| IBIS file generated by GenIBIS.pl Version 2.11
|   omap3530cbc
[IBIS ver]   4.1
[File name]   sprm323.ibs
[File Rev]   1.0
[Date]   Thu Dec 10, 2009, 9:15:0
[Source]   Data created at Texas Instruments
[Notes]   1) Model checked with IBISCHK4 and contains...
   16 errors relating to DC endpoints. These errors can be waived
   and relate to special modelling of active feedback IOs.
   180 warnings relating to non-monotonic behavior, non-zero
   GND/POWER Clamp values and C_comp max/min values. These
   warnings can be waived.
[Disclaimer] Please be aware that in the absence of a written agreement,
   Texas Instruments (TI) assumes no liability for: 1) the
   accuracy of the IBIS models provided to your company, 2) the
   proper functioning of these IBIS models in your design or for
   any resulting applications, or, 3) infringement of patents,
   copyrights, or intellectual property rights resulting from
   your use of these IBIS models. TI provides IBIS models as a
   service to our customers and therefore reserves the right to
   limit distribution of the IBIS models.
[Copyright]   Property of Texas Instruments Incorporated. Unauthorised
   reproduction and/or distribution is strictly prohibited. This
   product is protected under copyright law and trade secret law
   as an unpublished work. Created 1999,(C) Copyright 1999-2001,
   Texas Instruments Incorporated., All Rights Reserved. These
   commodities are under the U.S. Government distribution license
   control.As such,they are not to be re-exported without the
   prior approval of the U.S. Department of Commerce.
|   Component omap3530cbc
[Component]   omap3530cbc
[Manufacturer]   Texas Instruments.
[Package]
|   typ   min   max
R_pkg   1.24535   3.07E-2   2.46E0
L_pkg   4.9035E-009   3.77E-10   9.43E-9
C_pkg   1.941E-012   5.72E-13   3.31E-12
[Pin]   signal_name   model_name   R_pin   L_pin   C_pin
A3   gpmc_ncs2   Selector16   7.47E-1   2.93E-9   1.21E-12
A24   cam_d2   Selector12   6.25E-1   3.26E-9   1.31E-12
AA1   gpmc_d1   Selector16   1.96E0   8.19E-9   3.09E-12
AA2   gpmc_d0   Selector16   1.81E0   7.48E-9   3.08E-12
AA3   etk_d3   Selector16   6.29E-1   3.01E-9   1.20E-12
AA4   etk_d8   Selector1   8.17E-1   3.80E-9   1.32E-12
AA24   uart2_rts   Selector23   2.77E-1   2.00E-9   9.98E-13
AA25   dss_data12   Selector24   3.83E-1   1.97E-9   1.03E-12
AB1   etk_d5   Selector1   6.42E-1   3.90E-9   1.49E-12
AB2   etk_clk   Selector16   7.57E-1   3.49E-9   1.17E-12
AB4   i2c3_scl   Selector7   8.04E-1   3.18E-9   1.54E-12
AB25   dss_data23   Selector24   3.95E-1   2.43E-9   7.96E-13
AB26   dss_data15   Selector24   3.76E-1   2.32E-9   1.19E-12
AC1   gpmc_d3   Selector16   2.44E0   9.43E-9   3.17E-12
AC3   etk_d0   Selector16   7.48E-1   3.54E-9   1.20E-12
AC4   i2c3_sda   Selector7   4.25E-1   1.96E-9   1.16E-12
AC6   gpmc_nwp   Selector1   1.90E0   7.54E-9   3.00E-12
AC8   gpmc_wait1   Selector16   1.77E0   6.52E-9   2.93E-12
AC11   gpmc_wait0   Selector26   1.56E0   5.94E-9   2.85E-12
AC25   dss_data22   Selector24   3.90E-1   2.06E-9   9.02E-13
AC26   dss_data10   Selector24   4.20E-1   2.22E-9   1.12E-12
AD1   gpmc_ncs1   Selector16   2.18E0   9.09E-9   3.27E-12
AD3   etk_d2   Selector16   7.54E-1   3.54E-9   1.19E-12
AD5   gpmc_d6   Selector16   2.12E0   8.02E-9   3.26E-12
AD6   gpmc_d5   Selector16   1.82E0   7.47E-9   2.93E-12
AD7   sys_nreswarm   Selector25   5.19E-1   2.57E-9   2.06E-12
AD8   gpmc_ncs0   Selector11   1.84E0   6.93E-9   3.12E-12
AD16   gpio_113   Selector9   3.55E-1   1.79E-9   1.04E-12
AD17   gpio_112   Selector31   3.06E-1   1.92E-9   1.09E-12
AD21   uart2_rx   Selector23   2.39E-1   1.71E-9   9.84E-13
AD23   dss_data4   Model19   7.20E-1   2.65E-9   1.21E-12
AD24   dss_data5   Model19   6.03E-1   2.55E-9   1.08E-12
AD26   dss_data11   Selector24   4.78E-1   2.34E-9   1.08E-12
AE3   etk_d6   Selector1   9.02E-1   4.42E-9   1.31E-12
AE4   etk_d10   Selector1   8.76E-1   4.69E-9   1.67E-12
AE6   etk_d12   Selector1   7.45E-1   3.29E-9   1.36E-12
AE9   etk_d15   Selector1   4.16E-1   2.87E-9   1.34E-12
AE14   sys_clkout1   Selector5   7.36E-1   3.62E-9   1.65E-12
AE15   cam_d1   Selector3   1.92E-1   1.75E-9   9.80E-13
AE16   cam_d0   Selector20   1.57E-1   1.38E-9   9.16E-13
AE17   gpio_115   Selector32   3.17E-1   2.36E-9   1.04E-12
AE21   dss_data0   Model19   5.10E-1   2.83E-9   1.42E-12
AE23   dss_data2   Model19   4.99E-1   3.29E-9   1.11E-12
A23   cam_wen   Selector1   5.52E-1   3.42E-9   1.33E-12
AA26   dss_data14   Selector24   3.46E-1   1.74E-9   1.04E-12
AB3   etk_ctl   Selector16   6.33E-1   3.04E-9   1.35E-12
AC2   gpmc_d2   Selector16   2.46E0   8.74E-9   3.20E-12
AC5   gpmc_d7   Selector16   1.91E0   7.35E-9   3.03E-12
AD2   etk_d7   Selector1   8.44E-1   4.04E-9   1.21E-12
AD4   etk_d1   Selector1   8.44E-1   3.97E-9   1.36E-12
AD10   gpmc_nadv_ale   Selector22   1.79E0   7.57E-9   3.16E-12
AD15   i2c4_scl   Selector21   4.33E-1   2.80E-9   1.29E-12
AD22   uart2_tx   Selector23   3.75E-1   2.44E-9   1.11E-12
AE5   gpmc_d4   Selector16   1.96E0   7.81E-9   3.31E-12
AE18   gpio_114   Selector13   3.09E-1   2.36E-9   9.80E-13
AE20   sys_32k   Model94   1.18E0   6.31E-9   2.27E-12
AE22   dss_data1   Model19   4.68E-1   2.77E-9   1.32E-12
AE24   dss_data3   Model19   6.80E-1   3.18E-9   1.27E-12
AF6   etk_d11   Selector1   1.02E0   4.26E-9   1.32E-12
AF7   etk_d13   Selector1   1.17E0   5.30E-9   1.75E-12
AF9   etk_d14   Selector1   5.90E-1   3.89E-9   1.47E-12
AF19   sys_xtalin   Model82   7.18E-1   3.00E-9   1.26E-12
B3   gpmc_wait2   Selector16   7.66E-1   3.69E-9   1.31E-12
B4   gpmc_ncs4   Selector16   5.76E-1   3.21E-9   1.17E-12
B5   gpmc_ncs6   Selector16   6.68E-1   3.19E-9   1.21E-12
B6   gpmc_ncs3   Selector16   6.49E-1   2.82E-9   1.30E-12
B23   cam_fld   Selector1   4.18E-1   2.91E-9   1.11E-12
B24   cam_d3   Selector12   5.18E-1   2.76E-9   1.16E-12
C1   i2c2_sda   Selector7   1.72E0   6.60E-9   2.51E-12
C2   i2c2_scl   Selector7   1.54E0   6.33E-9   2.44E-12
C3   sys_boot2   Selector18   1.50E0   6.37E-9   2.20E-12
C4   gpmc_ncs5   Selector16   6.97E-1   3.53E-9   1.21E-12
C5   gpmc_ncs7   Selector16   4.85E-1   2.50E-9   1.27E-12
C6   gpmc_wait3   Selector16   4.60E-1   2.30E-9   1.21E-12
C23   cam_hs   Selector1   3.12E-1   2.16E-9   1.04E-12
C24   cam_d5   Selector12   5.71E-1   2.36E-9   1.16E-12
C25   cam_xclka   Selector1   5.14E-1   2.85E-9   1.05E-12
C26   cam_pclk   Selector1   5.65E-1   3.44E-9   1.23E-12
D1   gpmc_a9   Selector16   9.12E-1   4.13E-9   1.74E-12
D2   gpmc_a10   Selector16   5.01E-1   3.27E-9   1.44E-12
D3   sys_boot1   Selector18   1.64E0   6.91E-9   2.73E-12
D4   sys_boot6   Selector18   1.47E0   5.94E-9   2.63E-12
D23   cam_vs   Selector1   3.72E-1   2.45E-9   1.11E-12
D24   cam_d4   Selector12   4.53E-1   1.78E-9   1.04E-12
D25   cam_d10   Selector12   5.59E-1   2.67E-9   1.09E-12
D26   cam_strobe   Selector1   5.32E-1   3.02E-9   1.07E-12
E1   gpmc_a7   Selector16   7.35E-1   4.07E-9   1.41E-12
E2   gpmc_a8   Selector16   4.80E-1   3.15E-9   1.28E-12
E3   sys_boot3   Selector18   1.51E0   6.23E-9   2.64E-12
E4   sys_boot4   Selector18   1.35E0   5.60E-9   2.40E-12
E25   cam_xclkb   Selector1   4.33E-1   2.69E-9   9.49E-13
E26   cam_d11   Selector1   4.59E-1   2.76E-9   9.36E-13
F1   gpmc_a5   Selector1   8.42E-1   4.22E-9   1.51E-12
F2   gpmc_a6   Selector16   7.94E-1   3.87E-9   1.47E-12
F3   sys_boot0   Selector18   1.45E0   5.48E-9   2.37E-12
F23   uart3_cts_rctx   Selector23   3.29E-1   1.68E-9   1.11E-12
F24   uart3_rts_sd   Selector23   2.70E-1   1.77E-9   9.83E-13
F25   dss_data20   Selector2   5.35E-1   2.94E-9   9.30E-13
F26   dss_acbias   Selector8   5.81E-1   3.51E-9   1.15E-12
G2   gpmc_a4   Selector1   7.36E-1   4.12E-9   1.56E-12
G3   sys_boot5   Selector18   1.32E0   5.19E-9   2.07E-12
G24   uart3_tx_irtx   Selector23   3.45E-1   2.18E-9   1.00E-12
G25   dss_pclk   Selector2   3.63E-1   2.24E-9   8.87E-13
G26   dss_data6   Selector8   3.96E-1   2.81E-9   1.10E-12
H1   gpmc_a2   Selector1   1.04E0   4.79E-9   1.82E-12
H2   gpmc_a3   Selector1   8.67E-1   4.11E-9   1.60E-12
H3   uart1_rx   Selector1   1.06E0   3.86E-9   1.47E-12
H24   uart3_rx_irrx   Selector23   2.90E-1   1.95E-9   6.96E-13
H25   dss_data7   Selector8   4.05E-1   2.79E-9   9.14E-13
H26   dss_data8   Selector8   4.43E-1   2.90E-9   9.44E-13
J1   gpmc_nbe1   Selector1   1.12E0   5.06E-9   1.81E-12
J2   gpmc_a1   Selector1   1.01E0   4.83E-9   1.80E-12
J23   hdq_sio   Selector23   1.45E-1   1.42E-9   1.13E-12
J24   i2c1_sda   Selector4   3.24E-1   2.10E-9   9.83E-13
J25   i2c1_scl   Selector4   1.15E-1   1.35E-9   8.80E-13
J26   dss_data9   Selector8   4.62E-1   3.03E-9   9.58E-13
K2   gpmc_nbe0_cle   Selector1   9.96E-1   4.57E-9   1.82E-12
K3   mmc2_dat7   Selector1   1.24E0   6.44E-9   2.30E-12
K18   mmc1_dat2   Selector28   2.94E-1   2.34E-9   1.22E-12
K24   dss_hsync   Selector2   2.27E-1   1.57E-9   8.73E-13
L2   gpmc_d14   Selector16   3.82E-1   2.10E-9   1.19E-12
L3   mmc2_dat6   Selector1   6.40E-1   2.77E-9   1.14E-12
L4   uart1_tx   Selector10   6.79E-1   3.49E-9   1.88E-12
L18   mmc1_cmd   Selector28   2.79E-1   2.17E-9   9.60E-13
L25   dss_data16   Selector8   2.53E-1   1.30E-9   8.13E-13
L26   dss_data17   Selector8   4.54E-1   3.09E-9   1.09E-12
M1   gpmc_nwe   Selector11   4.67E-1   2.17E-9   1.19E-12
M2   gpmc_d15   Selector16   3.28E-1   1.78E-9   1.03E-12
M3   mmc2_dat5   Selector1   7.43E-1   4.22E-9   1.96E-12
M18   mmc1_dat1   Selector28   2.82E-1   1.81E-9   9.77E-13
M19   mmc1_dat0   Selector28   2.13E-1   1.61E-9   6.88E-13
M20   mmc1_dat4   Selector6   1.99E-1   1.66E-9   8.17E-13
M24   dss_data18   Selector8   3.27E-1   1.44E-9   8.69E-13
M25   dss_vsync   Selector2   3.10E-1   2.18E-9   1.10E-12
M26   dss_data19   Selector8   3.90E-1   2.24E-9   8.08E-13
N1   gpmc_clk   Selector1   7.04E-1   3.92E-9   1.73E-12
N2   gpmc_noe   Selector11   6.04E-1   2.69E-9   1.24E-12
N3   mcbsp3_dr   Selector1   5.26E-1   2.45E-9   1.07E-12
N19   mmc1_clk   Selector28   1.45E-1   1.74E-9   9.13E-13
N20   mmc1_dat3   Selector28   1.01E-1   1.19E-9   6.33E-13
N24   dss_data21   Selector8   4.35E-1   2.40E-9   9.99E-13
N25   cam_d8   Selector15   4.37E-1   2.49E-9   9.27E-13
N26   cam_d9   Selector17   3.55E-1   2.45E-9   9.81E-13
P1   gpmc_d13   Selector16   7.40E-1   4.30E-9   2.00E-12
P3   mcbsp3_dx   Selector1   4.51E-1   2.01E-9   9.47E-13
P7   mcspi1_somi   Selector14   4.61E-1   2.36E-9   1.03E-12
P8   mcspi1_simo   Selector14   3.00E-1   1.40E-9   7.95E-13
P9   mcspi1_clk   Selector14   3.47E-1   1.85E-9   7.54E-13
P17   mmc1_dat5   Selector6   3.28E-1   2.48E-9   1.39E-12
P18   mmc1_dat6   Selector6   2.59E-1   2.33E-9   9.77E-13
P19   mmc1_dat7   Selector6   1.89E-1   1.93E-9   7.54E-13
P20   mcbsp1_fsx   Selector1   2.37E-1   2.33E-9   9.07E-13
P25   cam_d6   Selector19   4.93E-1   1.98E-9   1.12E-12
P26   cam_d7   Selector30   4.82E-1   2.37E-9   8.33E-13
R2   uart1_rts   Selector10   3.09E-1   2.17E-9   9.35E-13
R3   mcbsp4_dx   Selector1   1.02E-1   1.66E-9   9.81E-13
R7   mcspi1_cs0   Selector14   2.61E-1   1.49E-9   6.48E-13
R8   mcspi1_cs1   Selector14   2.71E-1   1.44E-9   1.66E-12
R9   mcspi1_cs2   Selector14   3.46E-1   2.20E-9   9.66E-13
R10   mmc2_cmd   Selector16   4.22E-1   2.14E-9   8.09E-13
R18   mcbsp2_clkx   Selector14   2.60E-1   2.11E-9   8.58E-13
R19   mcbsp2_dx   Selector14   1.96E-1   1.82E-9   7.11E-13
T1   gpmc_d10   Selector16   1.14E0   5.46E-9   2.19E-12
T3   mcbsp4_fsx   Selector1   4.59E-1   2.81E-9   1.34E-12
T8   mcspi1_cs3   Selector16   3.46E-1   1.61E-9   1.72E-12
T9   mmc2_dat1   Selector16   4.08E-1   2.06E-9   8.68E-13
T10   mmc2_dat0   Selector16   3.34E-1   1.94E-9   8.12E-13
T17   mcbsp1_clkx   Selector1   3.41E-1   2.70E-9   9.99E-13
T18   mcbsp2_dr   Selector14   3.68E-1   2.37E-9   8.89E-13
T19   mcbsp_clks   Selector1   2.58E-1   1.71E-9   8.20E-13
T20   mcbsp1_dr   Selector1   2.70E-1   1.42E-9   6.81E-13
U1   gpmc_d12   Selector16   5.96E-1   3.80E-9   1.80E-12
U2   gpmc_d11   Selector16   1.27E0   5.73E-9   2.38E-12
U3   mcbsp3_clkx   Selector1   1.39E-1   1.67E-9   9.93E-13
U4   mcbsp4_dr   Selector12   2.59E-1   1.82E-9   1.04E-12
U8   mcspi2_somi   Selector1   6.06E-1   3.40E-9   1.49E-12
U9   mmc2_dat3   Selector16   4.96E-1   2.56E-9   1.08E-12
U10   mmc2_dat2   Selector16   5.08E-1   2.50E-9   1.16E-12
U15   jtag_ntrst   Selector27   6.11E-1   2.84E-9   8.87E-13
U16   jtag_tdi   Model71   5.29E-1   2.78E-9   8.93E-13
U17   mcbsp1_dx   Selector1   3.09E-1   2.47E-9   1.12E-12
U18   mcbsp2_fsx   Selector14   3.54E-1   2.31E-9   9.48E-13
U19   mcbsp1_clkr   Selector1   1.73E-1   1.70E-9   8.85E-13
U20   hsusb0_stp   Selector16   3.12E-1   1.58E-9   8.48E-13
V1   gpmc_d8   Selector16   1.46E0   6.54E-9   2.46E-12
V2   etk_d9   Selector1   3.29E-1   2.50E-9   8.29E-13
V3   mcbsp4_clkx   Selector1   3.99E-1   2.11E-9   9.74E-13
V8   mcspi2_cs0   Selector16   6.63E-1   3.57E-9   1.54E-12
V9   mcspi2_cs1   Selector1   6.34E-1   3.43E-9   1.61E-12
V10   mmc2_dat4   Selector1   5.69E-1   3.58E-9   1.27E-12
V12   sys_off_mode   Selector25   3.46E-1   2.02E-9   1.08E-12
V13   sys_nrespwron   Model75   4.08E-1   2.14E-9   1.23E-12
V14   jtag_tck   Selector27   5.65E-1   2.77E-9   1.19E-12
V15   jtag_tms_tmsc   Selector29   5.43E-1   2.65E-9   9.97E-13
V16   sys_nirq   Selector23   2.09E-1   1.36E-9   8.78E-13
V17   mcbsp1_fsr   Selector1   3.07E-1   2.49E-9   1.13E-12
V18   hsusb0_data2   Selector1   2.94E-1   2.26E-9   9.31E-13
V19   hsusb0_dir   Selector1   2.87E-1   2.14E-9   1.03E-12
V20   hsusb0_data0   Selector1   2.73E-1   1.93E-9   7.84E-13
W2   uart1_cts   Selector12   3.42E-1   2.38E-9   9.23E-13
W3   mcbsp3_fsx   Selector1   3.64E-1   2.41E-9   1.02E-12
W7   mcspi2_clk   Selector1   5.48E-1   3.09E-9   1.19E-12
W8   mcspi2_simo   Selector1   7.07E-1   3.59E-9   1.50E-12
W10   mmc2_clk   Selector1   7.12E-1   4.00E-9   1.41E-12
W11   sys_clkout2   Selector1   1.72E-1   1.25E-9   9.43E-13
W13   jtag_rtck   Selector5   3.45E-1   2.12E-9   1.05E-12
W15   sys_clkreq   Selector25   2.67E-1   1.84E-9   8.88E-13
W16   i2c4_sda   Selector21   4.99E-1   2.44E-9   1.05E-12
W17   hsusb0_data4   Selector1   3.42E-1   2.23E-9   9.95E-13
W18   hsusb0_nxt   Selector1   2.37E-1   2.31E-9   9.78E-13
W19   hsusb0_clk   Selector1   4.24E-1   2.66E-9   9.02E-13
W20   hsusb0_data3   Selector1   1.50E-1   1.53E-9   6.88E-13
Y1   gpmc_d9   Selector16   1.59E0   7.11E-9   2.51E-12
Y3   etk_d4   Selector1   2.31E-1   1.56E-9   1.06E-12
Y13   jtag_tdo   Selector5   2.38E-1   1.32E-9   7.11E-13
Y14   jtag_emu1   Selector23   3.98E-1   2.16E-9   1.04E-12
Y15   jtag_emu0   Selector23   3.66E-1   1.99E-9   1.18E-12
Y17   hsusb0_data7   Selector1   5.56E-1   3.27E-9   1.03E-12
Y18   hsusb0_data5   Selector1   3.07E-1   2.39E-9   8.93E-13
Y19   hsusb0_data6   Selector1   3.56E-1   2.10E-9   7.98E-13
Y20   hsusb0_data1   Selector1   2.07E-1   1.97E-9   8.03E-13
Y24   uart2_cts   Selector23   3.69E-1   2.25E-9   1.26E-12
Y25   dss_data13   Selector24   3.72E-1   1.81E-9   9.39E-13
| Device pads which are not required to be modeled. Included for completeness
|A18   vdds
|AB24   vdds_sdi
|AC7   vdds
|AC15   vdds
|AC18   vdds
|AC19   vss_dsi
|AC21   vdd_core
|AC24   vdds
|AD18   vdds_csi2
|AD20   vdds
|AE10   vdds
|AE19   cap_vdd_dsi
|AC16   vss_csi2
|AD19   vdds_dsi
|AF20   sys_xtalout   BQ0073VDDUS.4
|C11   vdds
|D5   vpp
|D9   vdds
|D13   vdd_mpu_iva
|D15   vdd_core
|E24   vdds
|G4   vdds
|G9   vdd_mpu_iva
|G11   vdd_core
|G12   vdd_mpu_iva
|G18   vdd_core
|H7   vdd_mpu_iva
|H20   vdd_core
|J15   vdds
|J18   vdds
|K11   vdd_mpu_iva
|L7   vdds
|L9   vdd_mpu_iva
|L19   vss_csib
|L20   vdds_csib
|L24   vdds
|M4   vdds
|M7   vdd_core
|M9   vdd_mpu_iva
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[Model Selector] Selector1
Model4 1.8V-I/O-X-SLOW
Model5 1.8V-I/O-X-FAST
Model6 1.8V-INPUT-PD-X
Model7 1.8V-INPUT-PI-X
Model8 1.8V-INPUT-PU-X
| Model selector for model set 1,2,3
|   Usage O#1.8V#PD/PI/PU##BQ0232CS_7LM
[Model Selector] Selector2
Model1 1.8V-I/O-PD-X
Model2 1.8V-I/O-PI-X
Model3 1.8V-I/O-PU-X
| Model selector for model set 10,9
|   Usage I#1.8V###CSI2PHY3LANE_7LM.8
[Model Selector] Selector3
Model10 1.8V-INPUT-X-X-GPI mode
Model9 1.8V-INPUT-X-X-LPRX Mode
| Model selector for model set 11,12
|   Usage IOOD#1.8V#PD/PI/PU##BQ0246S_7LM
[Model Selector] Selector4
Model11 1.8000V-I/O_OPEN_DRAIN-X-STANDARD
Model12 1.8000V-I/O_OPEN_DRAIN-X-LOWC
| Model selector for model set 13,14,15
|   Usage O#1.8V###BQ0253CS_7LM
[Model Selector] Selector5
Model13 1.8V-I/O-PD-X
Model14 1.8V-I/O-PI-X
Model15 1.8V-I/O-PU-X
| Model selector for model set 16,17,18
|   Usage IO#1.8V#PD/PI/PU##BQ0447S_7LM
[Model Selector] Selector6
Model16 1.8V-I/O-PD-X
Model17 1.8V-I/O-PI-X
Model18 1.8V-I/O-PU-X
| Model selector for model set 11,12,23,24
|   Usage IO#1.8V#PD/PI/PU##BQ0246S_7LM
|   IOOD#1.8V#PD/PI/PU##BQ0246S_7LM
[Model Selector] Selector7
Model11 1.8000V-I/O_OPEN_DRAIN-X-STANDARD
Model12 1.8000V-I/O_OPEN_DRAIN-X-LOWC
Model23 1.8000V-I/O-X-X
Model24 1.8000V-I/O-X-HIGHC
| Model selector for model set 20,21,22
|   Usage O#1.8V#PD/PI/PU##BQ0230CS_7LM
[Model Selector] Selector8
Model20 1.8V-I/O-PD-X
Model21 1.8V-I/O-PI-X
Model22 1.8V-I/O-PU-X
| Model selector for model set 25,26
|   Usage I#1.8V###CSI2PHY3LANE_7LM.4
[Model Selector] Selector9
Model25 1.8V-INPUT-X-X-LPRX Mode
Model26 1.8V-INPUT-X-X-GPI mode
| Model selector for model set 4,5
|   Usage O#1.8V#PD/PI/PU##BQ0267CS_7LM
[Model Selector] Selector10
Model4 1.8V-I/O-X-SLOW
Model5 1.8V-I/O-X-FAST
| Model selector for model set 27,28
|   Usage O#1.8V#PD/PI/PU##OQ0164CS_7LM
[Model Selector] Selector11
Model27 1.8V-3-STATE-X-SLOW
Model28 1.8V-3-STATE-X-FAST
| Model selector for model set 6,7,8
|   Usage I#1.8V#PD/PI/PU##BQ0267CS_7LM
[Model Selector] Selector12
Model6 1.8V-INPUT-PD-X
Model7 1.8V-INPUT-PI-X
Model8 1.8V-INPUT-PU-X
| Model selector for model set 29,30
|   Usage I#1.8V###CSI2PHY3LANE_7LM.5
[Model Selector] Selector13
Model29 1.8V-INPUT-X-X-LPRX Mode
Model30 1.8V-INPUT-X-X-GPI mode
| Model selector for model set 31,32,33,34,35,36,37,38,39,40,41,42
|   Usage O#1.8V#PD/PI/PU##BQOMAPPROGIOCSHYFBPB_7LM
[Model Selector] Selector14
Model31 1.8V-I/O-PD-DS00
Model32 1.8V-I/O-PD-DS11
Model33 1.8V-I/O-PD-DS10
Model34 1.8V-I/O-PD-DS01
Model35 1.8V-I/O-PI-DS11
Model36 1.8V-I/O-PI-DS10
Model37 1.8V-I/O-PI-DS01
Model38 1.8V-I/O-PI-DS00
Model39 1.8V-I/O-PU-DS00
Model40 1.8V-I/O-PU-DS11
Model41 1.8V-I/O-PU-DS10
Model42 1.8V-I/O-PU-DS01
| Model selector for model set 43,44,45
|   Usage I#1.8V#PD/PI/PU##CCPV2_7LM.3
[Model Selector] Selector15
Model43 1.8V-I/O-PD-X
Model44 1.8V-I/O-PI-X
Model45 1.8V-I/O-PU-X
| Model selector for model set 46,47,48,49,50
|   Usage IO#1.8V#PD/PI/PU##BQ0268CS_7LM
|   O#1.8V#PD/PU##BQ0268CS_7LM
[Model Selector] Selector16
Model46 1.8V-I/O-X-SLOW
Model47 1.8V-I/O-X-FAST
Model48 1.8V-INPUT-PD-X
Model49 1.8V-INPUT-PI-X
Model50 1.8V-INPUT-PU-X
| Model selector for model set 51,52,53
|   Usage I#1.8V#PD/PI/PU##CCPV2_7LM.4
[Model Selector] Selector17
Model51 1.8V-I/O-PD-X
Model52 1.8V-I/O-PI-X
Model53 1.8V-I/O-PU-X
| Model selector for model set 54,55,56
|   Usage IO#1.8V#PD/PI/PU##BQ0228CS_7LM
[Model Selector] Selector18
Model54 1.8V-I/O-PD-X
Model55 1.8V-I/O-PI-X
Model56 1.8V-I/O-PU-X
| Model selector for model set 57,58,59
|   Usage I#1.8V#PD/PI/PU##CCPV2_7LM.1
[Model Selector] Selector19
Model57 1.8V-I/O-PD-X
Model58 1.8V-I/O-PI-X
Model59 1.8V-I/O-PU-X
| Model selector for model set 60,61
|   Usage I#1.8V###CSI2PHY3LANE_7LM.7
[Model Selector] Selector20
Model60 1.8V-INPUT-X-X-LPRX Mode
Model61 1.8V-INPUT-X-X-GPI mode
| Model selector for model set 62,63,64,65
|   Usage IOOD#1.8V#PD/PI/PU##BQ0245S_7LM
|   O#1.8V#PD/PI/PU##BQ0245S_7LM
[Model Selector] Selector21
Model62 1.8000V-I/O_OPEN_DRAIN-X-STANDARD
Model63 1.8000V-I/O_OPEN_DRAIN-X-LOWC
Model64 1.8000V-I/O-X-X
Model65 1.8000V-I/O-X-HIGHC
| Model selector for model set 66,67
|   Usage O#1.8V#PD/PI/PU##OQ0163CS_7LM
[Model Selector] Selector22
Model66 1.8V-3-STATE-X-SLOW
Model67 1.8V-3-STATE-X-FAST
| Model selector for model set 68,69,70
|   Usage IO#1.8V#PD/PI/PU##BQ0226CS_7LM
[Model Selector] Selector23
Model68 1.8V-I/O-PD-X
Model69 1.8V-I/O-PI-X
Model70 1.8V-I/O-PU-X
| Model selector for model set 72,73,74
|   Usage IO#1.8V#PD/PI/PU##SDI2_7LM
[Model Selector] Selector24
Model72 1.8V-I/O-PD-X
Model73 1.8V-I/O-PU-X
Model74 1.8V-I/O-PI-X
| Model selector for model set 76,77,78
|   Usage IO#1.8V#PD/PI/PU##BQ0234CS_7LM
[Model Selector] Selector25
Model76 1.8V-I/O-PD-X
Model77 1.8V-I/O-PI-X
Model78 1.8V-I/O-PU-X
| Model selector for model set 79,80,81
|   Usage I#1.8V#PD/PI/PU##IQ0101CS_7LM
[Model Selector] Selector26
Model79 1.8V-INPUT-PD-X
Model80 1.8V-INPUT-PI-X
Model81 1.8V-INPUT-PU-X
| Model selector for model set 83,84,85
|   Usage I#1.8V###IQ0120CS_7LM
[Model Selector] Selector27
Model83 1.8V-INPUT-PD-X
Model84 1.8V-INPUT-PU-X
Model85 1.8V-INPUT-PI-X
| Model selector for model set 86,87,88
|   Usage IO#1.8V#PD/PI/PU##BQ0247S_7LM
|   IO#1.8V3.0V#PD/PI/PU##BQ0247S_7LM
[Model Selector] Selector28
Model86 1.8000V-I/O-PD-X
Model87 1.8000V-I/O-PI-X
Model88 1.8000V-I/O-PU-X
| Model selector for model set 95,96,97
|   Usage IO#1.8V###BQ0254CS_7LM
[Model Selector] Selector29
Model95 1.8V-I/O-PD-X
Model96 1.8V-I/O-PU-X
Model97 1.8V-I/O-PI-X
| Model selector for model set 91,92,93
|   Usage I#1.8V#PD/PI/PU##CCPV2_7LM.2
[Model Selector] Selector30
Model91 1.8V-I/O-PD-X
Model92 1.8V-I/O-PI-X
Model93 1.8V-I/O-PU-X
| Model selector for model set 89,90
|   Usage I#1.8V###CSI2PHY3LANE_7LM.3
[Model Selector] Selector31
Model89 1.8V-INPUT-X-X-LPRX Mode
Model90 1.8V-INPUT-X-X-GPI mode
| Model selector for model set 98,99
|   Usage I#1.8V###CSI2PHY3LANE_7LM.6
[Model Selector] Selector32
Model98 1.8V-INPUT-X-X-LPRX Mode
Model99 1.8V-INPUT-X-X-GPI mode
| Models and submodels in the file (99): Model1 (I/O), Model2 (I/O), Model3 (I/O), Model4 (I/O), Model5 (I/O), Model6 (Input), Model7 (Input), Model8 (Input), Model9 (Input), Model10 (Input), Model11 (I/O_open_drain), Model12 (I/O_open_drain), Model13 (I/O), Model14 (I/O), Model15 (I/O), Model16 (I/O), Model17 (I/O), Model18 (I/O), Model19 (I/O), Model20 (I/O), Model21 (I/O), Model22 (I/O), Model23 (I/O), Model24 (I/O), Model25 (Input), Model26 (Input), Model27 (3-state), Model28 (3-state), Model29 (Input), Model30 (Input), Model31 (I/O), Model32 (I/O), Model33 (I/O), Model34 (I/O), Model35 (I/O), Model36 (I/O), Model37 (I/O), Model38 (I/O), Model39 (I/O), Model40 (I/O), Model41 (I/O), Model42 (I/O), Model43 (I/O), Model44 (I/O), Model45 (I/O), Model46 (I/O), Model47 (I/O), Model48 (Input), Model49 (Input), Model50 (Input), Model51 (I/O), Model52 (I/O), Model53 (I/O), Model54 (I/O), Model55 (I/O), Model56 (I/O), Model57 (I/O), Model58 (I/O), Model59 (I/O), Model60 (Input), Model61 (Input), Model62 (I/O_open_drain), Model63 (I/O_open_drain), Model64 (I/O), Model65 (I/O), Model66 (3-state), Model67 (3-state), Model68 (I/O), Model69 (I/O), Model70 (I/O), Model71 (Input), Model72 (I/O), Model73 (I/O), Model74 (I/O), Model75 (Input), Model76 (I/O), Model77 (I/O), Model78 (I/O), Model79 (Input), Model80 (Input)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
